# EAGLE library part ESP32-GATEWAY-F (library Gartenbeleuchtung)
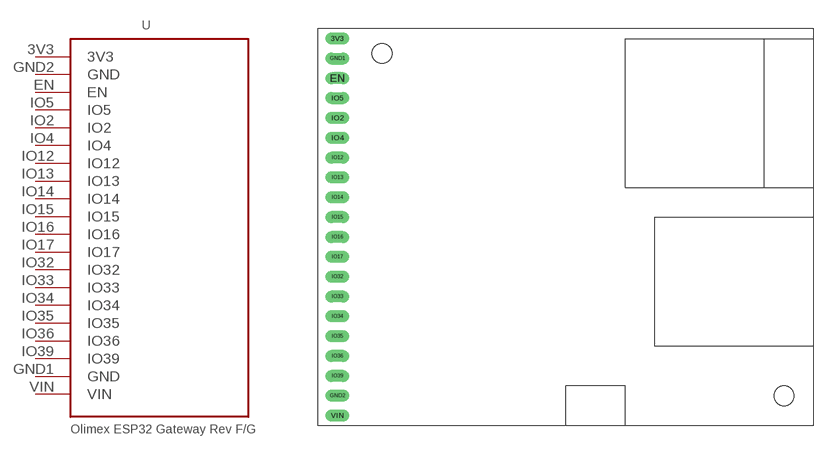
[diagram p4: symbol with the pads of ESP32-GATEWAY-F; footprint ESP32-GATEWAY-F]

Designator prefix -

## ESP32-GATEWAY-F  [ESP32-GATEWAY-F]
3V3  3V3  pwr
EN  EN
GND1  GND  pwr
GND2  GND  pwr
IO2  IO2
IO4  IO4
IO5  IO5
IO12  IO12
IO13  IO13
IO14  IO14
IO15  IO15
IO16  IO16
IO17  IO17
IO32  IO32
IO33  IO33
IO34  IO34
IO35  IO35
IO36  IO36
IO39  IO39
VIN  VIN  pwr

## Footprint ESP32-GATEWAY-F (pad centres in mm)
drill 1 pad 1.422 long: 3V3 0,0; EN 0,-5.08; GND1 0,-2.54; GND2 0,-45.72; IO2 0,-10.16; IO4 0,-12.7; IO5 0,-7.62; IO12 0,-15.24; IO13 0,-17.78; IO14 0,-20.32; IO15 0,-22.86; IO16 0,-25.4; IO17 0,-27.94; IO32 0,-30.48; IO33 0,-33.02; IO34 0,-35.56; IO35 0,-38.1; IO36 0,-40.64; IO39 0,-43.18; VIN 0,-48.26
